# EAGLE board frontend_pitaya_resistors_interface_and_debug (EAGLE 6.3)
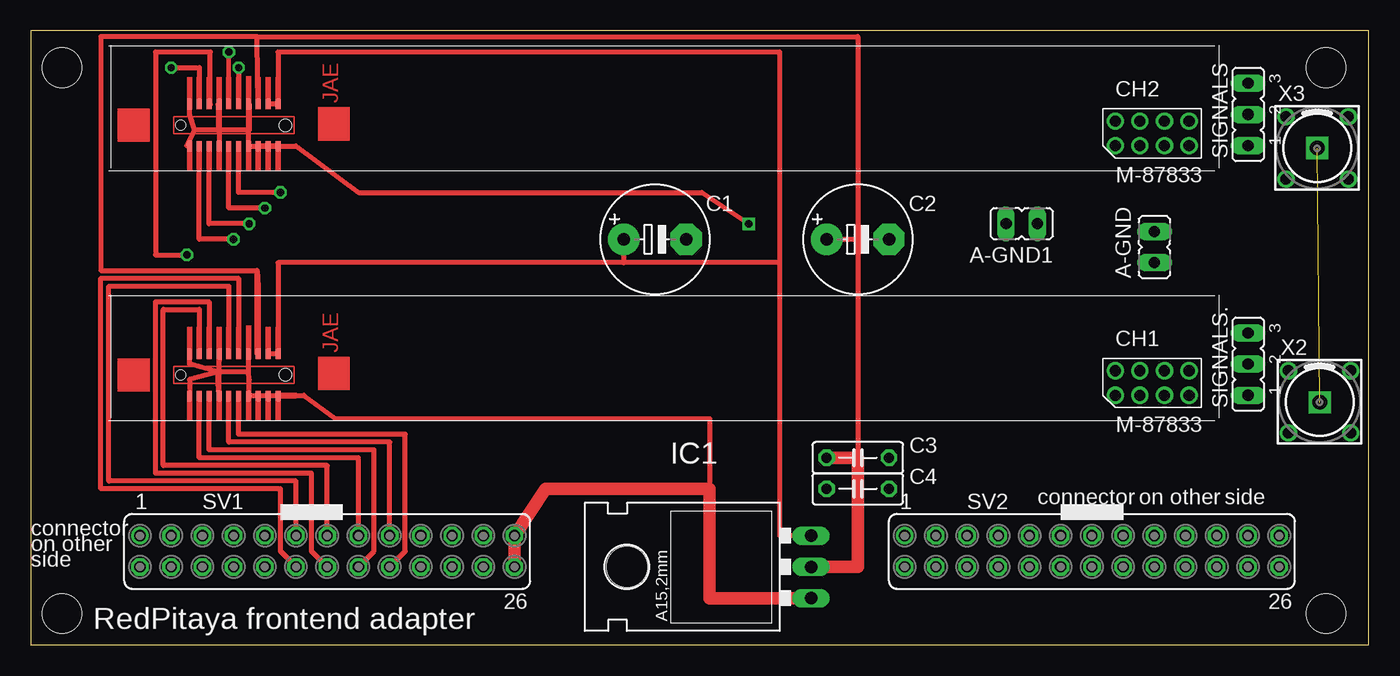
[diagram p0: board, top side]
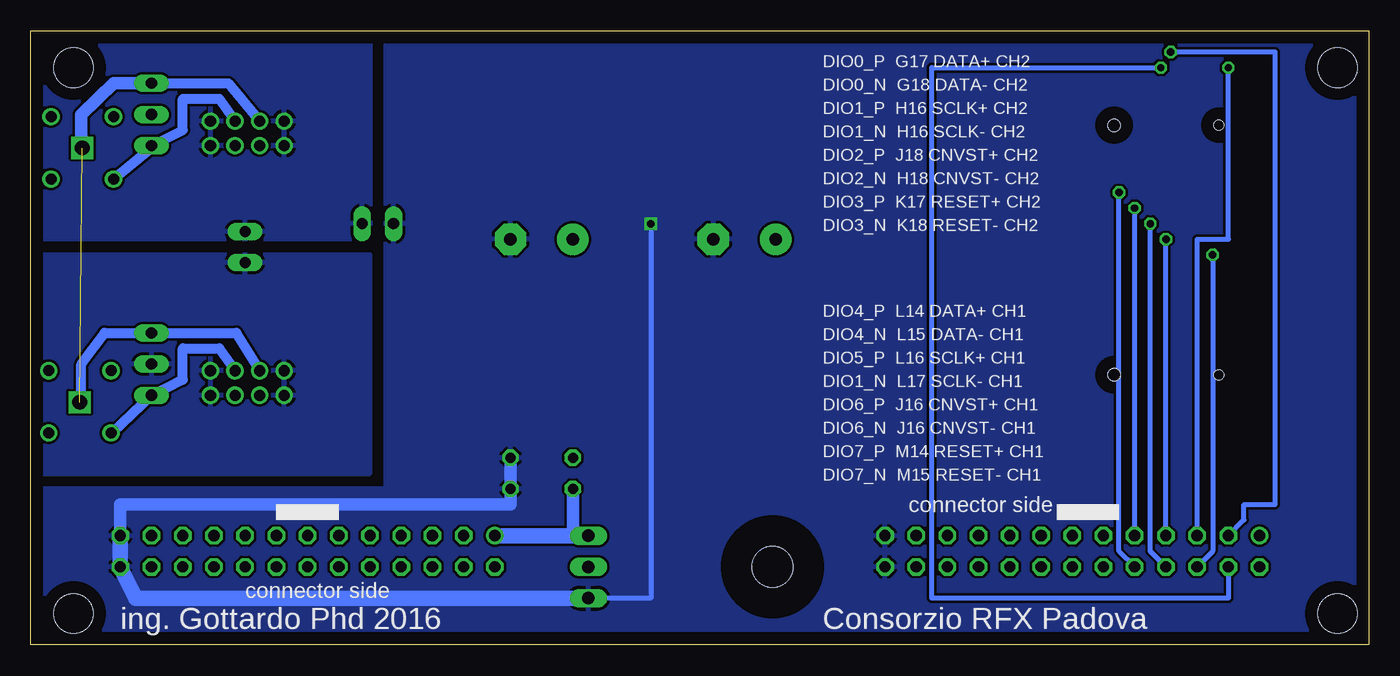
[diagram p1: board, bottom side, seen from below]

Size 108.89 x 50 mm. Coordinates in mm from the lower left corner, seen from the top.
Outline: 0,0 108.89,0 108.89,50 0,50 0,0
Copper layers (1*16): Top 0.035mm / dielectric 1.5mm / Bottom 0.035mm
Design rules "default": minimum track width 10mil, minimum drill 24mil, track to track 8mil, track to pad 8mil, pad to pad 8mil, via to via 8mil, smd to smd 8mil, copper to edge 40mil, drill to drill 8mil, minimum pad ring 10mil, minimum via ring 8mil, stop-mask expansion 4mil, vias tented up to drill 0mil, thermal gap 10mil
Holes 3.2 mm at 2.54,2.54 2.54,46.99 105.41,2.54 105.41,46.99

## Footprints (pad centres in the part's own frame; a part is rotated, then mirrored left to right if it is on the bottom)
JP1Y = drill 0.914 long: 1 0,-1.27; 2 0,1.27
E5-8,5 = drill 1.016 pad 2.54: + -2.54,0 | drill 1.016 pad 2.54 octagon: - 2.54,0
C050-025X075 = drill 0.813 octagon: 1 -2.54,0; 2 2.54,0
MOLEX87833 = drill 0.9: P$1 0,0; P$2 0,2; P$3 2,0; P$4 2,2; P$5 4,0; P$6 4,2; P$7 6,0; P$8 6,2
TO220L1 = drill 1.016 long: 1 -2.54,-3.81; 2 0,-3.81; 3 2.54,-3.81 | hole 3.302: 0,11.176
JP2 = drill 0.914 long: 1 -2.54,0; 2 0,0; 3 2.54,0
FE13-2 = drill 0.914: 1 -15.24,1.27 | drill 0.914 octagon: 2 -15.24,-1.27; 3 -12.7,1.27; 4 -12.7,-1.27; 5 -10.16,1.27; 6 -10.16,-1.27; 7 -7.62,1.27; 8 -7.62,-1.27; 9 -5.08,1.27; 10 -5.08,-1.27; 11 -2.54,1.27; 12 -2.54,-1.27; 13 0,1.27; 14 0,-1.27; 15 2.54,1.27; 16 2.54,-1.27; 17 5.08,1.27; 18 5.08,-1.27; 19 7.62,1.27; 20 7.62,-1.27; 21 10.16,1.27; 22 10.16,-1.27; 23 12.7,1.27; 24 12.7,-1.27; 25 15.24,1.27; 26 15.24,-1.27
JAECONNECTOR = smd 0.813 x 0.406: 3V3 0,5.6; 5VA 0,7.2; 5VB 0,6.4; A+ 3.4,3.2; A- 3.4,4; CV+ 3.4,0.8; CV- 3.4,1.6; G1 3.4,7.2; G3 3.4,6.4; G5 3.4,5.6; G7 3.4,4.8; G8 0,4.8; G13 3.4,2.4; G14 0,2.4; G19 3.4,0; G20 0,0; SC+ 0,0.8; SC- 0,1.6; SD+ 0,3.2; SD- 0,4 | hole 0.8: 1.7,7.9 | hole 1: 1.7,-0.6
EZG-00-302 = drill 0.6 pad 1: 1 0,-0.035; 2 -2.54,-2.505 | drill 0.9 pad 1.2: M1 -2.54,2.54; M2 2.54,2.54; M3 2.54,-2.54; M4 -2.54,-2.54

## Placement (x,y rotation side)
A-GND  bridge  [JP1Y]  91.44,32.38 0 top
A-GND1  bridge  [JP1Y]  80.64,34.29 90 top
C1  100uF  [E5-8,5]  50.8,33.02 0 top
C2  100uF  [E5-8,5]  67.31,33.02 0 top
C3  0.1uF  [C050-025X075]  67.31,15.24 0 top
C4  0.1uF  [C050-025X075]  67.31,12.7 0 top
CH1  MOLEX87833  [MOLEX87833]  88.27,20.32 0 top
CH2  MOLEX87833  [MOLEX87833]  88.27,40.64 0 top
IC1  LD1117AV  [TO220L1]  59.69,6.35 90 top
SIGNALS  [JP2]  99.06,43.18 90 top
SIGNALS.  [JP2]  99.06,22.86 90 top
SV1  [FE13-2]  24.13,7.62 0 top
SV2  [FE13-2]  86.36,7.62 0 top
U$5  JAE-CONNECTOR  [JAECONNECTOR]  20.12,40.6 90 top
U$6  JAE-CONNECTOR  [JAECONNECTOR]  20.12,20.29 90 top
X2  CH1  [EZG-00-302]  104.89,19.79 0 top
X3  CH2  [EZG-00-302]  104.69,40.46 0 top

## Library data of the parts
A-GND A-GND1 SIGNALS SIGNALS. = jumper
C1-C4 = resistor
CH1 CH2 = molex 87833
IC1 = v-reg
SV1 SV2 = con-lsta; OC_FARNELL: unknown; OC_NEWARK: unknown
U$5 U$6 = JAE-connector
X2 X3 = con-lemo

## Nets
GND: A-GND1.2 C1.- C2.- C3.2 C4.2 IC1.1 SV1.25 SV1.26 SV2.25 SV2.26 U$5.5VA U$5.G1 U$5.G7 U$5.G8 U$5.G13 U$5.G14 U$5.G20 U$5.SC+ U$5.SC- U$6.5VA U$6.G1 U$6.G7 U$6.G8 U$6.G13 U$6.G14 U$6.G20 U$6.SC+ U$6.SC-
N$2: C1.+ C4.1 IC1.3 SV2.1 U$5.CV+ U$5.G19 U$6.CV+ U$6.G19
S$1: CH1.P$6 SIGNALS..1 X2.2
S$2: CH1.P$4 SIGNALS..3 X2.1
S$3: A-GND1.1 A-GND.2 CH2.P$1 CH2.P$2 CH2.P$7 CH2.P$8
S$5: CH2.P$4 SIGNALS.3 X3.1
S$6: CH2.P$6 SIGNALS.1 X3.2
S$9: C2.+ C3.1 IC1.2 U$5.CV- U$6.CV-
S$10: SV1.13 U$6.G3
S$14: SV1.17 U$6.SD-
S$15: SV1.18 U$6.SD+
S$16: SV1.16 U$6.3V3
S$17: SV1.15 U$6.5VB
S$18: SV1.14 U$6.G5
S$19: SV1.11 U$6.A-
S$20: SV1.12 U$6.A+
S$21: SV1.10 U$5.SD+
S$22: SV1.9 U$5.SD-
S$23: SV1.8 U$5.3V3
S$24: SV1.7 U$5.5VB
S$25: SV1.5 U$5.G3
S$26: SV1.6 U$5.G5
S$27: SV1.3 U$5.A-
S$28: SV1.4 U$5.A+
S$33: A-GND.1 CH1.P$1 CH1.P$2 CH1.P$7 CH1.P$8 SIGNALS..2

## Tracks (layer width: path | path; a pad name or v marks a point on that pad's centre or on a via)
GND  (via drill 0.6)
  Top 0.406: 21.59,20.32 20.12,20.32 U$6.G20 | U$6.G20 21.59,20.29 21.59,20.32 | 21.59,20.32 22.23,20.32 24.77,18.41 55.24,18.41 55.24,12.7 | 12.92,23.5 U$6.G1 12.92,22.86 15.24,22.23 | U$6.G20 U$6.SC+ U$6.SC- | U$6.SC- 17.78,20.29 | 17.78,20.29 17.78,20.32 | 17.78,20.32 18.52,20.32 U$6.SC- | U$6.G14 17.78,20.29 | 17.78,20.32 17.78,21.59 17.72,22.23 | 17.72,22.23 15.32,22.23 | 15.32,22.23 U$6.G8 15.24,21.55 | 15.32,22.23 U$6.G7 15.24,21.14 15.24,21.55 | 17.72,22.23 U$6.G13 | 15.24,22.23 12.92,21.59 U$6.5VA | 15.24,21.55 15.24,22.23 | U$5.G20 U$5.SC+ U$5.SC- U$5.G14 | U$5.G14 U$5.G13 17.78,44.01 17.78,41.91 15.32,41.91 | 15.32,41.91 U$5.G7 15.24,44.01 15.24,41.91 13.34,41.91 | 15.32,41.91 U$5.G8 | 13.34,41.91 12.92,43.18 U$5.G1 | U$5.5VA 12.7,40.6 12.7,40.64 13.34,41.91 | U$5.G14 21.59,40.6 26.67,36.83 54.61,36.83 v58.42,34.29
  Top 1.016: IC1.1 55.24,3.81 55.24,12.7 41.91,12.7 SV1.25 SV1.26
  Bottom 0.406: v58.42,34.29 58.42,3.81 IC1.1
  Bottom 1.016: SV2.25 101.6,11.43 69.85,11.43 C4.2 C3.2
  Bottom 1.27: IC1.1 100.33,3.81 SV2.26 SV2.25
  pour Bottom: 0,50.8 80.01,50.8 80.01,12.7 110.49,12.7 110.49,-1.27 0,-1.27
N$2
  Top 0.406: 60.96,31.11 60.96,48.26 20.12,48.26 U$5.G19 U$5.CV+ | IC1.3 60.96,8.89 60.96,31.11 | 60.96,31.11 48.26,31.11 | 48.26,31.11 20.12,31.11 U$6.G19 U$6.CV+ | C1.+ 48.26,31.11
  Bottom 1.016: IC1.3 64.77,8.89 C4.1
  Bottom 1.27: SV2.1 IC1.3
S$1
  Bottom 0.406: X2.2 102.23,17.29
  Bottom 0.813: 102.23,17.29 SIGNALS..1 96.52,21.59 96.52,24.13 93.53,24.13 CH1.P$6
S$2
  Bottom 0.406: X2.1 104.78,19.75
  Bottom 0.813: 104.78,19.75 104.78,22.86 102.87,25.4 SIGNALS..3 92.17,25.4 CH1.P$4
S$3
  pour Bottom: 110.49,50.8 81.28,50.8 81.28,33.02 110.49,33.02
S$5  (via drill 1.2)  (2 unrouted)
  Bottom 0.813: SIGNALS.3 92.81,45.72 CH2.P$4
  Bottom 1.016: SIGNALS.3 102.15,45.72 104.78,43.18 104.78,40.42 X3.1
  other vias: 104.69,40.46 104.9,19.75
S$6
  Bottom 0.406: 99.06,40.49 SIGNALS.1
  Bottom 0.813: X3.2 99.06,40.49 | SIGNALS.1 96.52,41.91 96.52,44.45 93.53,44.45 CH2.P$6
S$9
  Top 0.406: U$5.CV- 18.41,49.09 18.41,49.53 | 18.41,49.53 5.71,49.53 5.71,30.48 18.41,30.48 | 18.41,30.48 18.41,23.68 U$6.CV- 18.52,29.21 18.41,30.48 | 18.41,49.53 67.31,49.53 67.31,33.02 | 67.31,33.02 67.31,15.24 | C2.+ 67.31,33.02
  Top 1.016: IC1.2 67.31,6.35 67.31,15.24 C3.1
S$10
  Top 0.406: SV1.13 24.13,14.61 10.79,14.61 10.79,27.3 13.72,27.3 U$6.G3
S$14
  Top 0.406: SV1.17 29.21,16.51 16.12,16.51 U$6.SD-
S$15
  Top 0.406: SV1.18 30.48,7.62 30.48,17.14 16.92,17.14 U$6.SD+
S$16
  Top 0.406: SV1.16 27.94,7.62 27.94,15.88 14.52,15.88 U$6.3V3
S$17
  Top 0.406: SV1.15 26.67,15.24 13.72,15.24 U$6.5VB
S$18
  Top 0.406: SV1.14 22.86,7.62 22.86,13.97 10.16,13.97 10.16,27.94 14.52,27.94 U$6.G5
S$19
  Top 0.406: SV1.11 21.59,13.34 6.35,13.34 6.35,29.21 16.12,29.21 U$6.A-
S$20
  Top 0.406: SV1.12 20.32,7.62 20.32,12.7 5.71,12.7 5.71,29.84 16.92,29.84 U$6.A+
S$21  (via drill 0.6)
  Top 0.406: v20.32,36.83 16.92,36.83 U$5.SD+
  Bottom 0.406: SV1.10 20.32,7.62 v20.32,36.83
S$22  (via drill 0.6)
  Top 0.406: v19.05,35.56 16.12,35.56 U$5.SD-
  Bottom 0.406: SV1.9 v19.05,35.56
S$23  (via drill 0.6)
  Top 0.406: v17.78,34.29 14.52,34.29 U$5.3V3
  Bottom 0.406: SV1.8 17.78,7.62 v17.78,34.29
S$24  (via drill 0.6)
  Top 0.406: v16.51,33.02 13.72,33.02 U$5.5VB
  Bottom 0.406: SV1.7 v16.51,33.02
S$25  (via drill 0.6)
  Top 0.406: v11.43,46.99 13.72,46.99 U$5.G3
  Bottom 0.406: SV1.5 13.97,33.02 11.43,33.02 v11.43,46.99
S$26  (via drill 0.6)
  Top 0.406: U$5.G5 14.61,44.01 14.61,48.26 10.16,48.26 10.16,31.75 v12.7,31.75
  Bottom 0.406: v12.7,31.75 12.7,7.62 SV1.6
S$27  (via drill 0.6)
  Top 0.356: v16.12,48.26 U$5.A-
  Bottom 0.406: SV1.3 10.16,10.16 10.16,11.43 7.62,11.43 7.62,48.26 v16.12,48.26
S$28  (via drill 0.6)
  Top 0.406: v16.92,46.99 U$5.A+
  Bottom 0.406: SV1.4 11.43,3.81 35.56,3.81 35.56,46.99 v16.92,46.99
S$33
  pour Bottom: 81.28,31.75 110.49,31.75 110.49,13.97 81.28,13.97

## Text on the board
tNames: connector | on other | side | connector | on other | side | RedPitaya frontend adapter
bNames: DIO0_P G17 DATA+ CH2 | DIO0_N G18 DATA- CH2 | DIO1_P H16 SCLK+ CH2 | DIO1_N H16 SCLK- CH2 | DIO2_P J18 CNVST+ CH2 | DIO2_N H18 CNVST- CH2 | DIO3_P K17 RESET+ CH2 | DIO3_N K18 RESET- CH2 | DIO4_P L14 DATA+ CH1 | DIO4_N L15 DATA- CH1 | DIO5_P L16 SCLK+ CH1 | DIO1_N L17 SCLK- CH1 | DIO6_P J16 CNVST+ CH1 | DIO6_N J16 CNVST- CH1 | DIO7_P M14 RESET+ CH1 | DIO7_N M15 RESET- CH1 | connector side | connector side | Consorzio RFX Padova | ing. Gottardo Phd 2016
